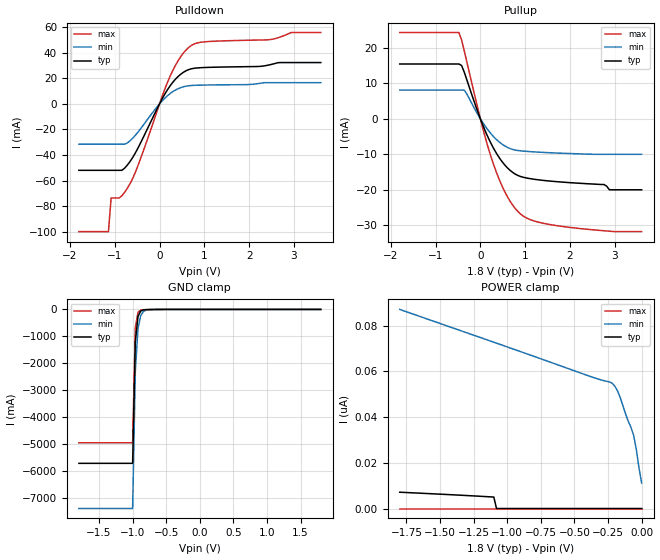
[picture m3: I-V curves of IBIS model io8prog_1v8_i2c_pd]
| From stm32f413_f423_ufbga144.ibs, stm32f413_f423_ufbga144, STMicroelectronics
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|   Model io8prog_1v8_i2c_pd
[Model]  io8prog_1v8_i2c_pd
Model_type I/O
Polarity   Non-Inverting
Enable   Active-Low
Vinl =   0.540000V
Vinh =   1.260000V
Vmeas =  0.900000V
Cref =   100.000000pF
Rref =   1.000000k
Vref =   1.800000V
C_comp   2.500900pF   2.333900pF   2.735800pF
[Temperature Range]   25.000000   0.125000k   -40.000000
[Pullup Reference]   1.800000V   1.600000V   2.000000V
[Pulldown Reference]   0.0V   0.0V   0.0V
[POWER Clamp Reference]   1.800000V   1.600000V   2.000000V
[GND Clamp Reference]   0.0V   0.0V   0.0V
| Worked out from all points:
|   slope of the pulldown table from 0 to 0.27 V, typ, clamps not added: 17.2 ohm
|   slope of the pullup table from 0 to 0.27 V, typ, clamps not added: 34.9 ohm
|   GND clamp passes 1 mA (typ) near -0.57 V on its own axis
[Pulldown]
|Voltage   I(typ)   I(min)   I(max)
-1.8V     -51.99mA   -31.53mA   -100mA
-1.14V    -51.99mA   -31.53mA   -100mA
-1.08V    -51.99mA   -31.53mA   -73.62mA
-900mV    -51.99mA   -31.53mA   -73.62mA
-660mV    -45.19mA   -28.93mA   -62.58mA
-480mV    -34.51mA   -22.06mA   -48.23mA
240mV     14.31mA    8.182mA    21.95mA
480mV     23.44mA    12.84mA    37.31mA
660mV     26.99mA    14.27mA    44.47mA
960mV     28.44mA    14.75mA    48.45mA
2.46V     30.61mA    16.66mA    50.32mA
3.6V      32.39mA    16.66mA    55.89mA
[Pullup]
|Voltage   I(typ)   I(min)   I(max)
-1.8V     15.46mA    8.103mA    24.33mA
-480mV    15.46mA    8.103mA    24.33mA
-360mV    13.15mA    8.103mA    19.18mA
60mV      -1.95mA    -1.198mA   -2.977mA
300mV     -8.441mA   -5.092mA   -13.07mA
600mV     -13.77mA   -8.025mA   -21.88mA
900mV     -16.27mA   -9.02mA    -26.86mA
1.2V      -17.03mA   -9.318mA   -28.8mA
1.74V     -17.74mA   -9.658mA   -30.18mA
2.76V     -18.51mA   -10mA      -31.55mA
2.88V     -20mA      -10mA      -31.68mA
3.6V      -20mA      -10mA      -31.8mA
[GND_clamp]
|Voltage   I(typ)   I(min)   I(max)
-1.8V     -5.722A    -7.401A    -4.956A
-1V       -5.722A    -7.401A    -4.956A
-960mV    -1.203A    -2.294A    -680.3mA
-920mV    -260.8mA   -717.4mA   -103.7mA
-880mV    -62.28mA   -228.9mA   -23.86mA
-840mV    -19.06mA   -76.33mA   -11.32mA
-760mV    -5.585mA   -11.67mA   -6.214mA
-640mV    -2.06mA    -2.422mA   -2.211mA
1.8V      44.31uA    33.68uA    51.4uA
[POWER_clamp]
|Voltage   I(typ)   I(min)   I(max)
-1.8V     7.131nA    87.08nA    0A
-1.1V     5.014nA    72.73nA    0A
-1.08V    0A         72.32nA    0A
-220mV    0A         54.8nA     0A
-200mV    0A         53.55nA    0A
-180mV    0A         51.5nA     0A
-160mV    0A         48.61nA    0A
-120mV    0A         41.45nA    0A
-60mV     0A         32.08nA    0A
-40mV     0A         25.93nA    0A
-20mV     0A         17.79nA    0A
0V        0A         11.13nA    0A
[Ramp]
| variable   typ   min   max
dV/dt_r  0.49514/6.00000u   0.27767/6.00000u   0.74652/6.00000u
dV/dt_f  0.75185/6.00000u   0.44015/6.00000u   0.96649/6.00000u
R_load = 50.000000
